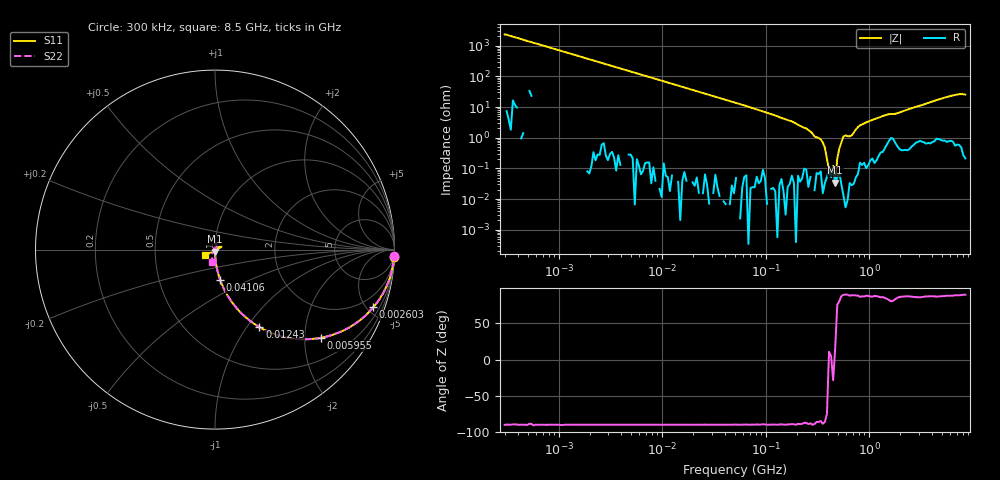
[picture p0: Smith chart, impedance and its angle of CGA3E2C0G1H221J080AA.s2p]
! S-parameter Generated by TDK Corporation
! Copyright(C) 2015 TDK Corporation.
! All Rights Reserved.
! TDK P/N: CGA3E2C0G1H221J080AA (Multilayer Ceramic Chip Capacitors)
! Property: C=220pF
! Size(LxWxT): 1.6x0.8x0.8mm, 0.063x0.031x0.031inches
! Model Type: s2p (Touchstone File Format Version 1.0)
! Frequency: DC=Yes Start=0.3MHz Stop=8500MHz 225points Log-sweep
! Note:
! Model Generated on Jun. 23, 2015
! Hash(MD5):
! Port Assignments:
!  1 ---| |--- 2
! Applicable Conditions:
!  Temperature = 25 degC
!  DC Bias Voltage = 0 V
!  Small Signal Operation
! Terms and conditions regarding TDK Simulation Models
! (1)This simulation model is being provided solely for informational purposes. Please refer to the specifications of the products in terms of detailed characteristics of such products.
! (2)In no event shall TDK Corporation of any of its subsidiaries be liable for any loss or damage arising, directly or indirectly,
!  From any information contained in this simulation model, including, but not limited to loss or damages arising from any inaccuracies, omissions or errors in connection with such information.
! (3)Any and all copyrights on this simulation model are owned by TDK Corporation.
!  Duplication or redistribution of this simulation model without prior written permission from TDK Corporation is prohibited.
! (4)This simulation model is subject to any modification or change without any prior notice.
! (5)Neither TDK Corporation nor any of its subsidiaries shall make any warranty, express or implied,
!  Including but not limited to the correctness, implied warranties of merchantability and fitness for a particular purpose with respect to this simulation models.
! (6)The use of this simulation model shall be deemed to have consented to the terms and conditions hereof.
# MHz S MA R 50
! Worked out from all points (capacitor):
!   224 points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, 300 kHz to 8.5 GHz, reference 50 ohm
!   read as one part in series: C = 224 pF near 314.1 kHz
!   lowest |Z| = 34 mohm at 469.5 MHz (marker M1)
!   series resonance near 407.6 MHz, so ESL is about 680 pH
!   S11 on the Smith chart (normalised r, x): 300 kHz: 1, -48; 2.603 MHz: 1.03, -5.49; 5.955 MHz: 1.00, -2.39; 12.43 MHz: 1.00, -1.15; 41.06 MHz: 1.00, -0.35; 8.5 GHz: 0.89, -0.05
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0.3  0.9991 -2.4  0.04314 87.9  0.04314 87.5  0.9991 -2.2
1.72111  0.9715 -13.6  0.2351 76.4  0.2346 76.3  0.9715 -13.6
2.603142  0.938 -20.0  0.3432 69.9  0.3432 69.9  0.9389 -20.0
5.954923  0.767 -39.9  0.6414 50.1  0.6411 50.2  0.7671 -39.9
9.430415  0.6026 -53.0  0.798 37.0  0.798 37.0  0.6026 -53.0
12.42578  0.4977 -60.2  0.8671 29.7  0.867 29.8  0.4972 -60.2
41.06062  0.1711 -80.3  0.9851 9.6  0.9852 9.6  0.1711 -80.3
51.67171  0.1364 -82.3  0.9902 7.7  0.9892 7.6  0.1361 -82.3
283.1228  0.02211 -89.1  0.9998 0.3  0.9998 0.3  0.02211 -90.3
469.456  0.01157 -84.9  0.9998 -0.7  0.9992 -0.6  0.01107 -94.4
778.4218  0.004965 -81.8  1 -2.8  0.9975 -2.8  0.005032 -102.5
1025.67  0.0008908 -112.6  0.9983 -4.1  0.9971 -4.1  0.003084 -15.0
1073.923  0.0003736 -124.3  0.9974 -4.4  0.9972 -4.4  0.003164 -3.0
1232.735  0.001077 18.1  0.9953 -5.1  0.9982 -5.1  0.002907 21.0
1551.304  0.006272 9.0  0.9911 -6.6  0.992 -6.6  0.008569 1.0
2346.313  0.003524 -51.2  0.9956 -9.8  0.995 -9.6  0.005825 -56.2
3389.298  0.008174 0.8  0.9931 -13.9  0.9914 -13.9  0.005284 9.0
4465.833  0.02299 34.0  0.9901 -18.4  0.99 -18.5  0.01959 60.5
6450.987  0.0391 24.1  0.9894 -26.5  0.9901 -26.6  0.0331 86.8
7404.957  0.02711 19.0  0.9905 -30.3  0.9886 -30.3  0.01975 96.9
7753.325  0.01109 -10.0  0.9903 -31.6  0.9919 -31.7  0.007014 159.0
8500  0.06169 -153.4  0.9882 -34.5  0.991 -34.5  0.06854 -103.9
